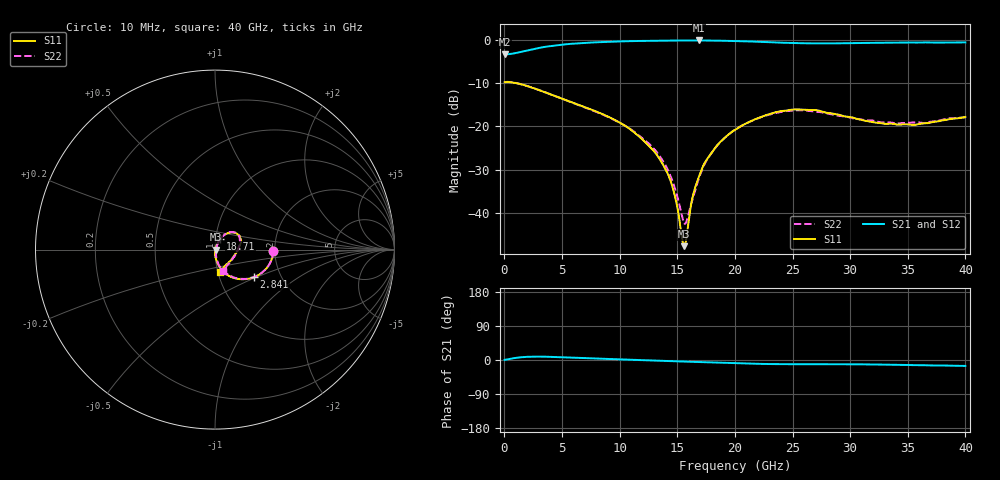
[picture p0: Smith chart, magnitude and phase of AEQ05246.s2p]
! Sonnet Data File
! From: emgraph Version : 16.52
! From Emgraph Data: AEQ05246_Sample
! Data File Written: 02/28/2018 11:53:21
!< HDATE 02/28/2018 11:50:43
!< MDATE 02/28/2018 11:50:43
# GHZ S MA R 50.00000
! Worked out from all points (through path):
!   6401 points, 10 MHz to 40 GHz, reference 50 ohm
!   highest |S21| = -0.20 dB at 16.87 GHz (marker M1); lowest = -3.4 dB at 10 MHz (marker M2)
!   group delay of S21, straight-line fit = 1.76 ps
!   lowest |S11| = -47.7 dB at 15.6 GHz (marker M3), VSWR 1.01, Z = 50.4 - j0.0609 ohm
!   |S11| at or under -10 dB: 933.4 MHz to end of sweep
!   |S22| runs from -42.5 to -9.8 dB; largest |S21 - S12| = 0.0041
!   S11 on the Smith chart (normalised r, x): 10 MHz: 1.95, -0.02; 2.841 GHz: 1.46, -0.48; 18.71 GHz: 1.05, +0.13; 40 GHz: 1.02, -0.26
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0.01  0.322 -0.9  0.6755 0.3  0.6787 0.4  0.3236 -1.3
2.840542  0.2662 -35.1  0.7939 9.0  0.7939 9.0  0.2661 -34.9
6.677083  0.1718 -60.7  0.9107 5.4  0.9109 5.4  0.1711 -59.4
10.68858  0.09691 -76.0  0.9576 1.0  0.9577 0.9  0.0974 -74.5
12.10698  0.06763 -81.5  0.9663 -0.6  0.9665 -0.6  0.0702 -77.9
13.34417  0.04432 -86.1  0.9713 -1.8  0.9711 -1.9  0.04782 -80.8
14.08148  0.03 -87.8  0.9731 -2.6  0.9734 -2.6  0.03333 -80.2
14.54387  0.02063 -88.7  0.9748 -3.0  0.9746 -3.1  0.02412 -77.3
14.96876  0.01219 -83.4  0.9759 -3.5  0.9758 -3.6  0.01608 -69.1
15.43114  0.004825 -45.2  0.976 -4.0  0.9763 -4.0  0.00889 -40.6
15.59985  0.004134 -8.4  0.9764 -4.1  0.9769 -4.2  0.007576 -19.0
15.7873  0.00516 30.9  0.9762 -4.3  0.9767 -4.4  0.007929 7.4
16.32467  0.01522 64.4  0.976 -4.8  0.9759 -4.9  0.0144 48.3
16.87453  0.02623 69.5  0.977 -5.4  0.9776 -5.5  0.02517 63.5
17.55561  0.04142 67.6  0.9747 -6.2  0.9754 -6.3  0.04074 65.1
18.70532  0.06556 65.0  0.9706 -7.4  0.9707 -7.5  0.06507 63.5
20.005  0.09112 59.2  0.9628 -8.6  0.9624 -8.7  0.09136 59.0
23.65409  0.1466 39.6  0.9253 -10.9  0.9251 -11.0  0.1432 42.9
26.67208  0.1539 20.9  0.9046 -11.0  0.9037 -11.2  0.1487 21.8
33.33917  0.1068 -31.0  0.9211 -12.4  0.92 -12.6  0.1109 -28.9
35.6011  0.1038 -54.1  0.9247 -13.6  0.9231 -13.8  0.1106 -46.7
40  0.128 -78.4  0.9282 -15.6  0.9245 -15.7  0.1266 -68.6
